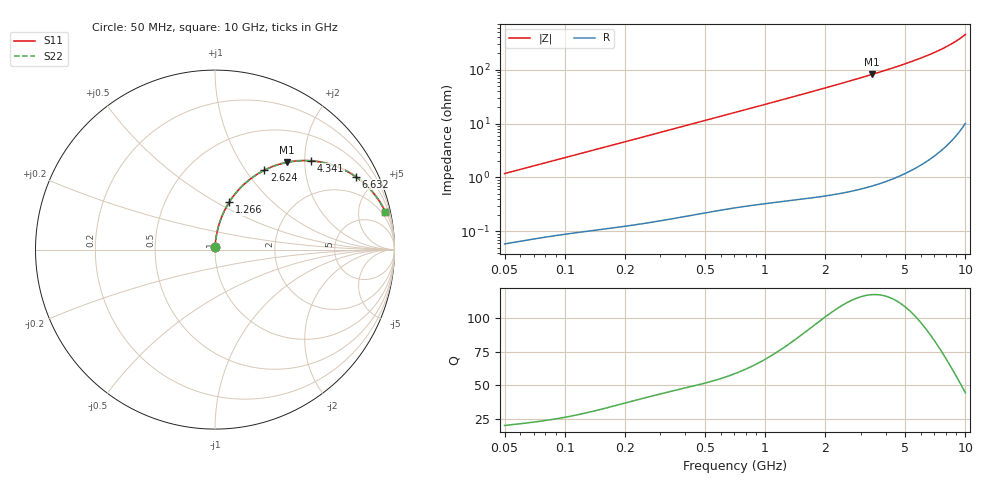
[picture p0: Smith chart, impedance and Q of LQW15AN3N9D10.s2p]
!Murata Part Number: LQW15AN3N9D10
!These Parameters are Measured in Series Mode Connection
!  o--[Z]--o
!Port1  Port2
!  o-------o
!Freq. Start=50[MHz] Stop=10[GHz], 401[Steps]
# Hz S RI R 50
!Freq.(Hz)	S 11(Real)	S 11(Imag)	S 21(Real)	S 21(Imag)	S 12(Real)	S 12(Imag)	S 22(Real)	S 22(Imag)
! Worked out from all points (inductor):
!   401 points, 50 MHz to 10 GHz, reference 50 ohm
!   read as one part in series: L = 3.74 nH near 51.34 MHz
!   highest Q = 118 at 3.42 GHz (marker M1), where L = 3.8 nH
!   S11 on the Smith chart (normalised r, x): 50 MHz: 1.00, +0.02; 1.266 GHz: 1.01, +0.58; 2.624 GHz: 1.01, +1.22; 4.341 GHz: 1.02, +2.16; 6.632 GHz: 1.04, +3.83; 10 GHz: 1.20, +9.00
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5e7  0.000725 0.0118  0.9993 -0.0118  0.9993 -0.0118  0.000725 0.0118
1.214486e8  0.00176 0.0281  0.9982 -0.0281  0.9982 -0.0281  0.00176 0.0281
1.956524e8  0.00325 0.0448  0.9968 -0.0448  0.9968 -0.0448  0.00325 0.0448
2.949953e8  0.00608 0.0671  0.9939 -0.0671  0.9939 -0.0671  0.00608 0.0671
4.689809e8  0.0134 0.1053  0.9866 -0.1053  0.9866 -0.1053  0.0134 0.1053
7.071068e8  0.0277 0.1559  0.9723 -0.1559  0.9723 -0.1559  0.0277 0.1559
9.717327e8  0.0493 0.2093  0.9507 -0.2093  0.9507 -0.2093  0.0493 0.2093
1.26648e9  0.0795 0.2643  0.9205 -0.2643  0.9205 -0.2643  0.0795 0.2643
1.717543e9  0.1364 0.3379  0.8636 -0.3379  0.8636 -0.3379  0.1364 0.3379
2.122994e9  0.1954 0.3918  0.8046 -0.3918  0.8046 -0.3918  0.1954 0.3918
2.624158e9  0.2742 0.4417  0.7258 -0.4417  0.7258 -0.4417  0.2742 0.4417
3.420121e9  0.4014 0.486  0.5986 -0.486  0.5986 -0.486  0.4014 0.486
4.171863e9  0.5138 0.4955  0.4862 -0.4955  0.4862 -0.4955  0.5138 0.4955
4.34098e9  0.5373 0.4943  0.4627 -0.4943  0.4627 -0.4943  0.5373 0.4943
4.826234e9  0.6008 0.4852  0.3992 -0.4852  0.3992 -0.4852  0.6008 0.4852
5.365732e9  0.664 0.4676  0.336 -0.4676  0.336 -0.4676  0.664 0.4676
6.632392e9  0.7828 0.4067  0.2172 -0.4067  0.2172 -0.4067  0.7828 0.4067
7.37379e9  0.8354 0.3645  0.1646 -0.3645  0.1646 -0.3645  0.8354 0.3645
8.198065e9  0.8817 0.3156  0.1183 -0.3156  0.1183 -0.3156  0.8817 0.3156
8.876195e9  0.9118 0.2751  0.0882 -0.2751  0.0882 -0.2751  0.9118 0.2751
9.738562e9  0.9414 0.2246  0.0586 -0.2246  0.0586 -0.2246  0.9414 0.2246
1e10  0.9487 0.2096  0.0513 -0.2096  0.0513 -0.2096  0.9487 0.2096
